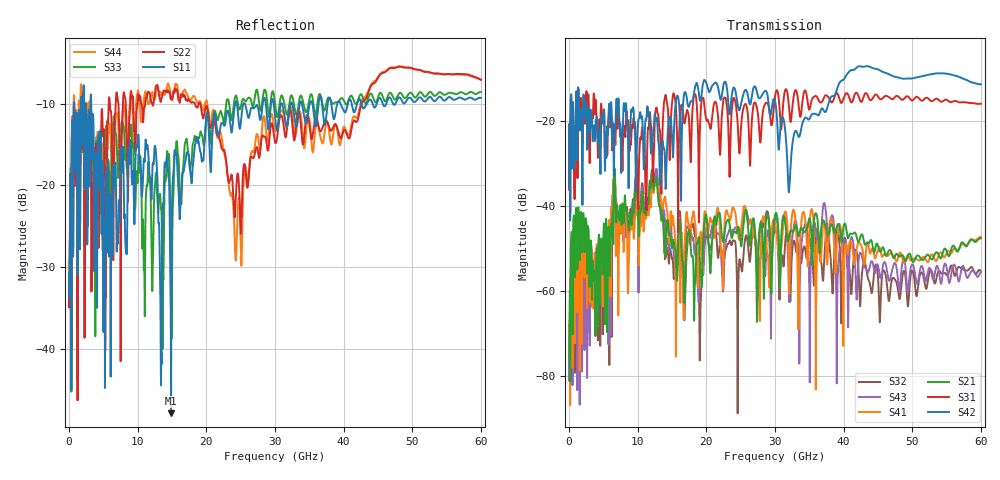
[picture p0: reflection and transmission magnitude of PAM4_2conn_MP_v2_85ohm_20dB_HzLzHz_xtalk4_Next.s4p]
! Info: Touchstone file created by Circ.  Input file=FAB50GbE_2conn_Midplane_Examax_Topo2_v2_85ohm_20dB_HzLzHz.circ
# Hz S RI R 50
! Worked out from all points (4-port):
!   6000 points, 10 MHz to 60 GHz, reference 50 ohm
!   strongest paths, dB at 10 MHz, 15.01 GHz, 30.01 GHz, 45.01 GHz, 60 GHz:
!     S42: -35.5, -24.0, -15.3, -7.9, -11.4
!     S31: -36.2, -15.7, -14.2, -14.2, -16.0
!     S21: -75.4, -49.8, -42.2, -49.4, -47.6
!     S41: -68.0, -44.3, -43.8, -50.4, -47.3
!     S43: -71.0, -48.5, -43.1, -53.9, -55.5
!     S32: -74.7, -52.5, -45.3, -56.8, -55.4
!   lowest |S11| = -47.9 dB at 14.86 GHz (marker M1), VSWR 1.01, Z = 50.3 - j0.246 ohm
!   |S11| at or under -10 dB: 3.231 GHz to 24.21 GHz (20.98 GHz wide, 153 % of centre); 25.62 GHz to 28.22 GHz (2.603 GHz wide, 9.67 % of centre); 31.01 GHz to 32.28 GHz (1.267 GHz wide, 4 % of centre)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
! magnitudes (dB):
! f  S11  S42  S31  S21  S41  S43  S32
! 10 MHz  -33.6  -35.5  -36.2  -75.4  -68.0  -71.0  -74.7
! 860 MHz  -17.6  -24.7  -24.0  -56.7  -66.3  -64.0  -67.3
! 6.6 GHz  -20.1  -24.1  -24.5  -32.3  -31.1  -32.5  -34.1
! 14.86 GHz  -47.9  -20.1  -19.0  -48.0  -41.4  -44.2  -51.2
! 24.27 GHz  -9.8  -13.2  -15.8  -46.2  -42.1  -45.0  -49.2
! 32.06 GHz  -11.2  -36.5  -17.1  -47.3  -60.6  -61.8  -52.7
! 60 GHz  -9.3  -11.4  -16.0  -47.6  -47.3  -55.5  -55.4
